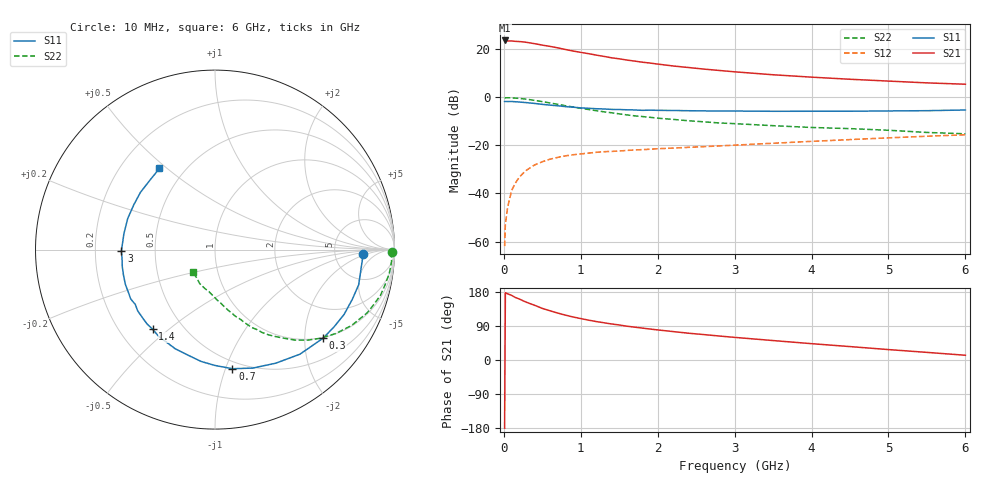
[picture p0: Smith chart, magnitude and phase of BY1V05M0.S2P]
! SIEMENS Small Signal Semiconductors
! BFY420
! Si NPN RF SIEGET Grounded Emitter Transistor in MICRO-X
! VCE = 1 V  IC = 5 mA
! Common Emitter S-Parameters:  October  1996
# GHz  S  MA  R  50
!  f  S11  S21  S12  S22
! GHz  MAG  ANG  MAG  ANG  MAG  ANG  MAG  ANG
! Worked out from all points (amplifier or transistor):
!   36 points, 10 MHz to 6 GHz, reference 50 ohm
!   highest |S21| = 23.7 dB at 10 MHz (marker M1)
!   |S21| within 3 dB of that: start of sweep to 687.7 MHz
!   unconditionally stable (mu >= 1): 3.07 GHz to end of sweep
!   at 250 MHz: K = 0.12, MSG = 27.4 dB, |S12| = -31.6 dB
!   at 1.4 GHz: K = 0.55, MSG = 19.5 dB, |S12| = -22.5 dB
!   at 6 GHz: K = 1.16, MAG = 8.1 dB, |S12| = -15.6 dB
!   S11 on the Smith chart (normalised r, x): 10 MHz: 10, -1; 300 MHz: 0.98, -2.46; 700 MHz: 0.44, -1.06; 1.4 GHz: 0.34, -0.44; 3 GHz: 0.31, -0.01; 6 GHz: 0.36, +0.47
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0.01  0.8259 -1.6  15.38 -179.9  0.0008 100.3  0.9878 -0.8
0.02  0.8242 -2.9  15.34 177.6  0.0023 89.9  0.982 -1.5
0.05  0.8208 -6.8  15.04 174.6  0.0052 86.8  0.986 -3.8
0.1  0.8243 -13.7  15.01 170.7  0.0114 84.5  0.9801 -7.8
0.15  0.8136 -19.9  14.75 164.9  0.0165 78.8  0.9677 -11.7
0.2  0.8048 -26.7  14.59 161.1  0.0217 76.1  0.9567 -15.4
0.25  0.7907 -33.0  14.38 156.3  0.0263 72.0  0.9361 -19.1
0.3  0.7788 -39.3  14.01 151.9  0.031 69.3  0.918 -22.6
0.4  0.7507 -50.9  13.2 144.4  0.0393 63.8  0.8703 -29.1
0.5  0.7179 -61.8  12.3 136.2  0.0458 58.8  0.8191 -34.8
0.6  0.6929 -72.3  11.58 129.9  0.0518 54.5  0.7684 -40.0
0.7  0.6707 -81.7  10.8 123.9  0.0565 50.9  0.7202 -44.5
0.9  0.6276 -97.2  9.27 113.5  0.0641 44.9  0.6319 -51.6
1.1  0.5953 -111.8  8.175 105.2  0.0694 40.9  0.5618 -57.8
1.4  0.5637 -128.0  6.702 95.1  0.0751 36.8  0.4801 -64.7
1.7  0.5494 -141.7  5.718 86.7  0.0807 34.7  0.414 -69.9
2.2  0.5356 -158.8  4.526 75.0  0.0883 32.1  0.3495 -77.3
3  0.5216 -179.1  3.419 59.7  0.1016 30.2  0.2848 -86.8
3.5  0.5152 170.0  2.969 51.3  0.1113 28.8  0.2584 -92.3
4.5  0.5168 151.0  2.393 35.4  0.1326 24.5  0.2243 -104.5
5.5  0.5304 132.9  2.012 20.1  0.1558 18.4  0.1868 -123.6
6  0.5481 124.4  1.886 12.5  0.1669 14.9  0.175 -135.7
